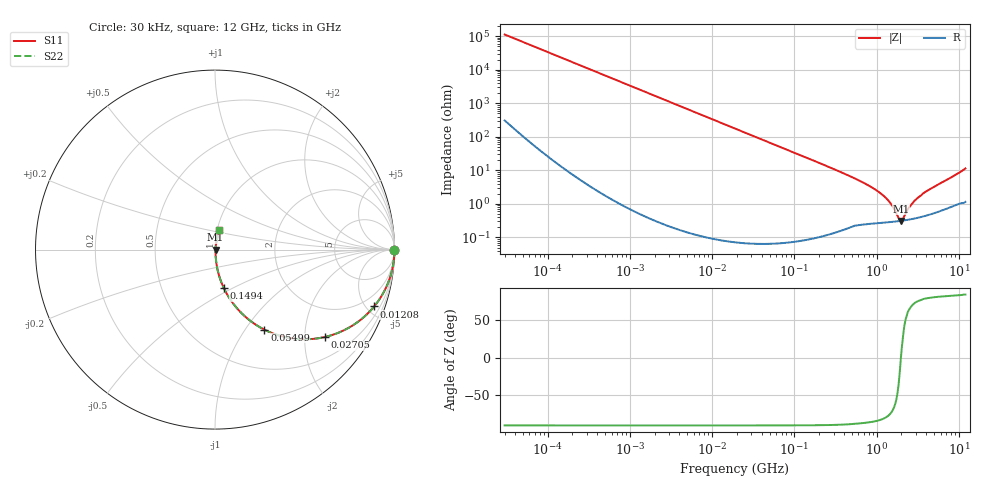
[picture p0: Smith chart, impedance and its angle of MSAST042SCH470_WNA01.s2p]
! MSAST042SCH470_WNA01  S-PARAMETER MODEL  ( General Type )
! Model Generated by TAIYO YUDEN Corporation (http://www.ty-top.com)
! Version 1.0
! TAIYO YUDEN Control No. 150820
! Copyright(c) 2015 TAIYO YUDEN CO.,LTD. All Rights Reserved.
! Product Description (link to TY-COMPAS)
! https://ds.yuden.co.jp/TYCOMPAS/or/detail?pn=MSAST042SCH470JWNA01&u=M
! Products Name : Multilayer Ceramic Capacitors
! Characteristics :
!  Capacitance : 47 pF , Rated Voltage : 25V , TCC : CH / C0H
!  Case Size : 0.4 x 0.2 / 0.016 x 0.008 [mm/inch] , Thickness : 0.2 / 0.008 [mm/inch]
!  (Conditions: Temperature = 25 degC , DC Bias Current/Voltage = 0A / 0V)
! External Node Assignments :
!  1  o---| |---o  2
! GND o---------o GND
! Frequency Range : 0.03MHz  -  12000MHz  [ 401 STEP ]
# MHz S RI R 50
! Freq[MHz].  S11 Real  S11 Imag  S21 Real  S21 Imag  S12 Real  S12 Imag  S22 Real  S22 Imag
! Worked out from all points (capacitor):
!   401 points, 30 kHz to 12 GHz, reference 50 ohm
!   read as one part in series: C = 47 pF near 32 kHz
!   lowest |Z| = 313 mohm at 1.972 GHz (marker M1)
!   series resonance near 1.973 GHz, so ESL is about 140 pH
!   S11 on the Smith chart (normalised r, x): 30 kHz: open; 12.08 MHz: 1.00, -5.61; 27.05 MHz: 1.00, -2.50; 54.99 MHz: 1.00, -1.23; 149.4 MHz: 1.00, -0.45; 12 GHz: 1.02, +0.23
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0.03  1 -0.000886  3.21e-06 0.000886  3.21e-06 0.000886  1 -0.000886
0.260295  0.9999 -0.00769  6.19e-05 0.00769  6.19e-05 0.00769  0.9999 -0.00769
2.258455  0.9956 -0.0664  0.00444 0.0664  0.00444 0.0664  0.9956 -0.0664
5.39449  0.9752 -0.1554  0.0248 0.1554  0.0248 0.1554  0.9752 -0.1554
12.08034  0.887 -0.3164  0.113 0.3164  0.113 0.3164  0.887 -0.3164
18.97367  0.7609 -0.4263  0.2391 0.4263  0.2391 0.4263  0.7609 -0.4263
27.05253  0.6103 -0.4874  0.3897 0.4874  0.3897 0.4874  0.6103 -0.4874
38.57132  0.4351 -0.4954  0.5649 0.4954  0.5649 0.4954  0.4351 -0.4954
54.99475  0.2748 -0.4459  0.7252 0.4459  0.7252 0.4459  0.2748 -0.4459
86.37604  0.1332 -0.3389  0.8668 0.3389  0.8668 0.3389  0.1332 -0.3389
149.4448  0.0491 -0.214  0.9509 0.214  0.9509 0.214  0.0491 -0.214
164.6252  0.0409 -0.1957  0.9591 0.1957  0.9591 0.1957  0.0409 -0.1957
749.4426  0.00396 -0.0384  0.996 0.0384  0.996 0.0384  0.00396 -0.0384
1103.571  0.00315 -0.021  0.9969 0.021  0.9969 0.021  0.00315 -0.021
1428.372  0.00299 -0.0112  0.997 0.0112  0.997 0.0112  0.00299 -0.0112
1573.464  0.00299 -0.00777  0.997 0.00777  0.997 0.00777  0.00299 -0.00777
1848.769  0.00307 -0.0022  0.9969 0.0022  0.9969 0.0022  0.00307 -0.0022
1971.936  0.00312 -9.94e-06  0.9969 9.94e-06  0.9969 9.94e-06  0.00312 -9.94e-06
2103.309  0.0032 0.00188  0.9968 -0.00188  0.9968 -0.00188  0.0032 0.00188
2722.352  0.00365 0.00983  0.9963 -0.00983  0.9963 -0.00983  0.00365 0.00983
3639.072  0.00457 0.0197  0.9954 -0.0197  0.9954 -0.0197  0.00457 0.0197
12000  0.0237 0.1097  0.9763 -0.1097  0.9763 -0.1097  0.0237 0.1097
